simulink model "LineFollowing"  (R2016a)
settings: Solver=VariableStepDiscrete  StartTime=0.0  StopTime=inf  RelTol=1e-3
model workspace (MAT data in the model file):
  MCOS : class17 (value not decoded)
  MCOS : class17 (value not decoded)
  MCOS : class17 (value not decoded)
  MCOS : class17 (value not decoded)
  MCOS : class17 (value not decoded)
  MCOS : class17 (value not decoded)
undefined symbols (not defined in the file or in its folder): axleLength, commandPercmPerSecond, sampleTime, symmetrizeMotors
libraries: miniQ x2, simulink x1

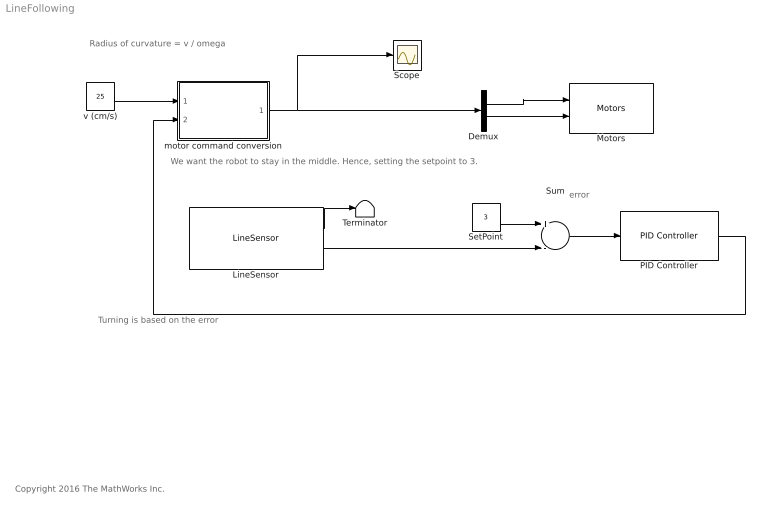
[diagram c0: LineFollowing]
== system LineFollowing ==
  note: Copyright 2016 The MathWorks Inc.
  note: Turning is based on the error
  note: error
  note: We want the robot to stay in the middle. Hence, setting the setpoint to 3.
  note: Radius of curvature = v / omega
  Demux : Demux  Outputs=2
  LineSensor : miniQ/LineSensor  sampleTime_dd=0.01  maxRawSensors=[800,900,900,900,800]  minRawSensors=[200,280,300,300,220]  debug_dd=off
  Motors : miniQ/Motors  flipLeft=off  flipRight=off
  PID Controller : simulink/Continuous/PID Controller  Controller=PID  TimeDomain=Discrete-time  SampleTime=-1  IntegratorMethod=Forward Euler  FilterMethod=Forward Euler  Form=Parallel  UseFilter=on  ControllerParametersSource=internal  P=10  I=0  D=0.005  N=1  InitialConditionSource=internal  InitialConditionForIntegrator=0  InitialConditionForFilter=0  ExternalReset=none  LimitOutput=off  UpperSaturationLimit=5  LowerSaturationLimit=-5  LinearizeAsGain=on  AntiWindupMode=none  Kb=1  TrackingMode=off  Kt=1  PParamMin=[]  PParamMax=[]  IParamMin=[]  IParamMax=[]  DParamMin=[]  DParamMax=[]  NParamMin=[]  NParamMax=[]  KbParamMin=[]  KbParamMax=[]  KtParamMin=[]  KtParamMax=[]  POutMin=[]  POutMax=[]  IOutMin=[]  IOutMax=[]  DOutMin=[]  DOutMax=[]  NOutMin=[]  NOutMax=[]  KbOutMin=[]  KbOutMax=[]  KtOutMin=[]  KtOutMax=[]  IntegratorOutMin=[]  IntegratorOutMax=[]  FilterOutMin=[]  FilterOutMax=[]  SumOutMin=[]  SumOutMax=[]  SumI1OutMin=[]  SumI1OutMax=[]  SumI2OutMin=[]  SumI2OutMax=[]  SumI3OutMin=[]  SumI3OutMax=[]  SumDOutMin=[]  SumDOutMax=[]  SaturationOutMin=[]  SaturationOutMax=[]  IntegratorContinuousStateAttributes=''  IntegratorStateMustResolveToSignalObject=off  IntegratorRTWStateStorageClass=Auto  FilterContinuousStateAttributes=''  FilterStateMustResolveToSignalObject=off  FilterRTWStateStorageClass=Auto  DifferentiatorICPrevScaledInput=0  DifferentiatorOutMin=[]  DifferentiatorOutMax=[]
  Scope : Scope
  SetPoint : Constant  Value=3
  Sum : Sum  Inputs=+-
  Terminator : Terminator
  motor command conversion : Subsystem
  v (cm/s) : Constant  Value=25  SampleTime=sampleTime
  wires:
  v (cm/s)/1 -> motor command conversion/1(v)
  motor command conversion/1(v_L v_R) -> Scope/1, Demux/1
  Demux/1 -> Motors/1
  Demux/2 -> Motors/2
  LineSensor/1 -> Terminator/1
  LineSensor/2 -> Sum/2
  SetPoint/1 -> Sum/1
  Sum/1 -> PID Controller/1
  PID Controller/1 -> motor command conversion/2(omega)

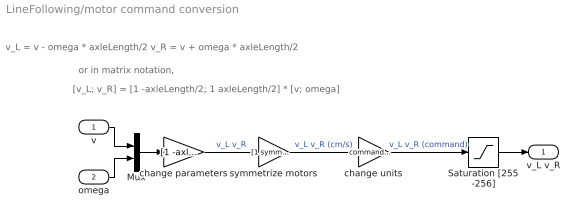
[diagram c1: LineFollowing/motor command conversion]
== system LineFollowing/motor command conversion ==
  note: or in matrix notation,
  note: v_L = v - omega * axleLength/2 v_R = v + omega * axleLength/2
  note: [v_L; v_R] = [1 -axleLength/2; 1 axleLength/2] * [v; omega]
  v : Inport
  omega : Inport  Port=2
  Mux : Mux  Inputs=2
  Saturation [255 -256] : Saturate  UpperLimit=255  LowerLimit=-256
  change parameters : Gain  Gain=[1 -axleLength/2; 1 axleLength/2]  Multiplication=Matrix(K*u)
  change units : Gain  Gain=commandPercmPerSecond
  symmetrize motors : Gain  Gain=[1 symmetrizeMotors]
  v_L v_R : Outport
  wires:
  change parameters/1 -> symmetrize motors/1  "v_L v_R"
  change units/1 -> Saturation [255 -256]/1  "v_L v_R (command)"
  symmetrize motors/1 -> change units/1  "v_L v_R (cm/s)"
  Saturation [255 -256]/1 -> v_L v_R/1
  Mux/1 -> change parameters/1
  omega/1 -> Mux/2
  v/1 -> Mux/1
